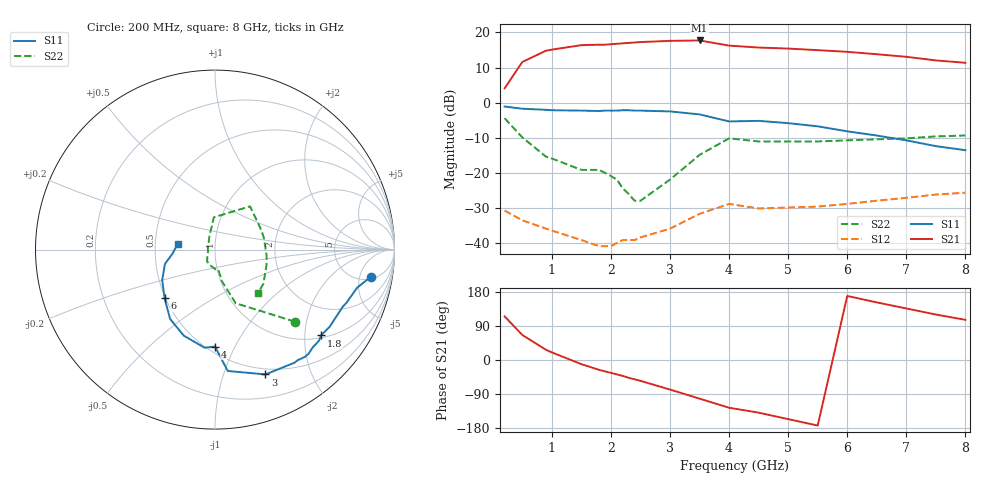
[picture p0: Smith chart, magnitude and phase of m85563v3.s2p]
!MGA-85563 S PARAMETERS
!Vd=3V LAST UPDATED 05-29-97
# ghz s ma r 50
!FREQ  S11  S21  S12  S22
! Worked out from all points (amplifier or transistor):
!   24 points, 200 MHz to 8 GHz, reference 50 ohm
!   highest |S21| = 17.7 dB at 3.5 GHz (marker M1)
!   |S21| within 3 dB of that: 890.4 MHz to 5.745 GHz (4.854 GHz wide, 146 % of centre)
!   unconditionally stable (mu >= 1): start of sweep to end of sweep
!   at 1.5 GHz: K = 2.81, MAG = 20.4 dB, |S12| = -39.2 dB
!   at 2.5 GHz: K = 2.39, MAG = 21.3 dB, |S12| = -38.4 dB
!   at 8 GHz: K = 2.22, MAG = 12.3 dB, |S12| = -25.7 dB
!   lowest NFmin = 1.56 dB at 1.8 GHz
!   S11 on the Smith chart (normalised r, x): 200 MHz: 5.48, -7.43; 1.8 GHz: 1.07, -2.41; 3 GHz: 0.44, -1.39; 4 GHz: 0.55, -0.84; 6 GHz: 0.49, -0.32; 8 GHz: 0.65, +0.04
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0.2  0.88 -10.0  1.6 115.0  0.029 1.0  0.6 -42.0
0.5  0.82 -15.0  3.8 66.0  0.021 -18.0  0.32 -69.0
0.9  0.79 -22.0  5.5 27.0  0.016 -16.0  0.17 -79.0
1  0.78 -24.0  5.7 20.0  0.015 -15.0  0.16 -78.0
1.5  0.77 -34.0  6.6 -11.0  0.011 -8.0  0.11 -81.0
1.8  0.76 -39.0  6.7 -26.0  0.009 5.0  0.11 -88.0
2.1  0.77 -45.0  6.9 -38.0  0.01 31.0  0.08 -123.0
2.2  0.78 -48.0  7 -42.0  0.011 34.0  0.06 -136.0
2.3  0.78 -50.0  7.1 -47.0  0.011 37.0  0.05 -149.0
2.4  0.77 -53.0  7.2 -51.0  0.011 39.0  0.04 -164.0
2.5  0.77 -55.0  7.3 -55.0  0.012 42.0  0.04 176.0
3  0.75 -68.0  7.6 -78.0  0.016 57.0  0.08 113.0
3.5  0.68 -84.0  7.7 -102.0  0.026 61.0  0.18 92.0
4  0.54 -90.0  6.5 -126.0  0.036 38.0  0.31 51.0
4.5  0.55 -96.0  6.1 -139.0  0.031 27.0  0.28 26.0
5  0.51 -110.0  5.9 -156.0  0.032 29.0  0.28 15.0
5.5  0.46 -123.0  5.6 -173.0  0.033 26.0  0.28 4.0
6  0.39 -136.0  5.3 169.0  0.036 25.0  0.29 -7.0
6.5  0.34 -150.0  4.9 152.0  0.04 23.0  0.3 -17.0
7  0.29 -164.0  4.5 136.0  0.044 19.0  0.31 -26.0
7.5  0.24 -174.0  4 120.0  0.049 14.0  0.33 -35.0
8  0.21 172.0  3.7 106.0  0.052 8.0  0.34 -45.0
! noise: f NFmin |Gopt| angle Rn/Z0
0.2  1.63  0.7  28  0.86
0.9  1.6  0.63  29  0.73
1.8  1.56  0.56  32  0.59
2  1.56  0.56  34  0.58
2.3  1.56  0.54  39  0.53
2.5  1.56  0.53  42  0.51
4  1.57  0.49  61  0.41
5  1.59  0.43  78  0.32
6.5  1.65  0.25  104  0.23
8  1.7  0.04  -48  0.15
